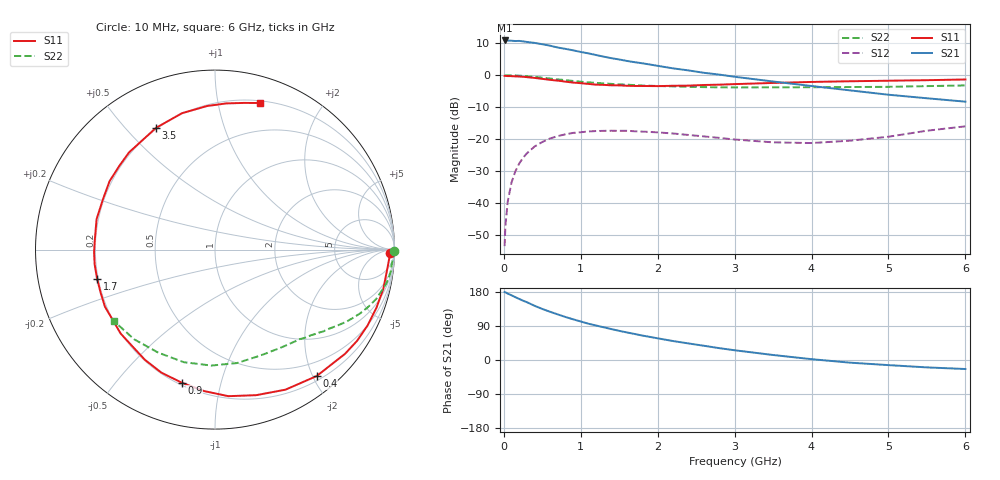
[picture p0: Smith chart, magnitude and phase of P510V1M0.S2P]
! SIEMENS Small Signal Semiconductors
! BFP183
! Si NPN RF Bipolar Junction Transistor in SOT143
! VCE = 10 V  IC = 1 mA
! Common Emitter S-Parameters:  March  1996
# GHz  S  MA  R  50
!  f  S11  S21  S12  S22
! GHz  MAG  ANG  MAG  ANG  MAG  ANG  MAG  ANG
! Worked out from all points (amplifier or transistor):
!   36 points, 10 MHz to 6 GHz, reference 50 ohm
!   highest |S21| = 10.8 dB at 10 MHz (marker M1)
!   |S21| within 3 dB of that: start of sweep to 881.1 MHz
!   unconditionally stable (mu >= 1): 2.534 GHz to end of sweep
!   at 250 MHz: K = 0.09, MSG = 18.2 dB, |S12| = -25.9 dB
!   at 1.4 GHz: K = 0.53, MSG = 11.4 dB, |S12| = -17.4 dB
!   at 6 GHz: K = 1.02, MAG = 2.9 dB, |S12| = -16.0 dB
!   S11 on the Smith chart (normalised r, x): 10 MHz: 46, -35; 400 MHz: 0.27, -2.06; 900 MHz: 0.21, -0.76; 1.7 GHz: 0.20, -0.12; 3.5 GHz: 0.19, +0.61; 6 GHz: 0.22, +1.33
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0.01  0.9726 -1.2  3.487 179.3  0.0021 84.1  0.9989 -0.4
0.02  0.9726 -2.7  3.467 178.7  0.0043 84.6  0.9906 -0.9
0.05  0.9654 -6.8  3.476 175.3  0.0104 87.8  0.9953 -2.2
0.1  0.9629 -13.3  3.451 170.7  0.0209 82.3  0.9882 -4.5
0.2  0.9493 -26.5  3.43 161.1  0.0413 73.9  0.9807 -9.0
0.3  0.9285 -38.7  3.304 152.5  0.0597 66.6  0.9602 -13.2
0.4  0.904 -51.2  3.193 143.0  0.0763 59.1  0.9394 -17.0
0.5  0.8736 -63.3  3.042 134.7  0.0898 52.3  0.9105 -20.6
0.6  0.8429 -74.2  2.891 127.3  0.1018 46.1  0.8833 -23.7
0.7  0.82 -84.8  2.703 120.4  0.1109 40.6  0.8573 -26.4
0.8  0.7903 -94.5  2.577 113.6  0.1183 35.5  0.8345 -28.8
0.9  0.7642 -104.1  2.444 107.4  0.1245 31.0  0.81 -31.1
1.1  0.7276 -122.5  2.189 95.7  0.1311 22.9  0.7701 -35.1
1.4  0.6917 -145.3  1.839 81.5  0.1346 12.9  0.7286 -40.3
1.7  0.6767 -166.2  1.594 68.7  0.1321 5.9  0.6967 -45.2
1.9  0.674 -178.5  1.464 60.9  0.1289 1.9  0.681 -48.2
2.2  0.6812 165.6  1.275 50.0  0.1219 -2.4  0.6651 -53.2
2.8  0.7083 138.8  1.019 31.3  0.1041 -5.3  0.6443 -64.2
3.5  0.7538 115.8  0.794 13.2  0.0886 0.6  0.6439 -79.0
4.5  0.8011 93.2  0.577 -7.0  0.0941 19.5  0.6509 -105.5
5.5  0.8328 78.9  0.434 -19.5  0.1348 27.3  0.6727 -132.0
6  0.8545 72.9  0.384 -23.8  0.1578 24.8  0.6895 -144.6
